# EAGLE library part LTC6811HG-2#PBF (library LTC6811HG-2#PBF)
Multicell Battery Balancer Automotive 48-Pin SSOP Tube Source: Datasheet
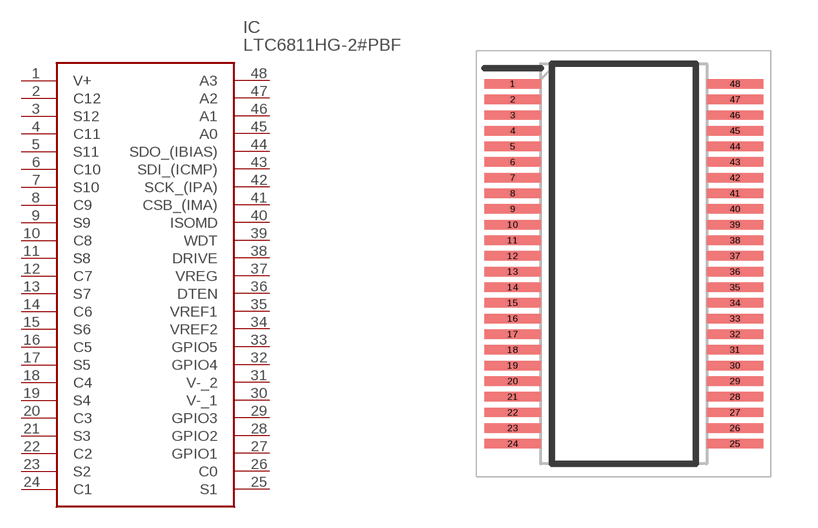
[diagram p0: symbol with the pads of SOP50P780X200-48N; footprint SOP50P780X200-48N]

Designator prefix IC

## LTC6811HG-2#PBF (Description: Multicell Battery Balancer Automotive 48-Pin SSOP Tube; Height: 2mm; Manufacturer_Name: Analog Devices; Manufacturer_Part_Number: LTC6811HG-2#PBF; Mouser_Part_Number: 584-LTC6811HG-2#PBF; Mouser_Price-Stock: https://www.mouser.co.uk/ProductDetail/Analog-Devices/LTC6811HG-2PBF?qs=oahfZPh6IAIAIIgZWv9WxQ%3D%3D)  [SOP50P780X200-48N]
1  V+
2  C12
3  S12
4  C11
5  S11
6  C10
7  S10
8  C9
9  S9
10  C8
11  S8
12  C7
13  S7
14  C6
15  S6
16  C5
17  S5
18  C4
19  S4
20  C3
21  S3
22  C2
23  S2
24  C1
25  S1
26  C0
27  GPIO1
28  GPIO2
29  GPIO3
30  V-_1
31  V-_2
32  GPIO4
33  GPIO5
34  VREF2
35  VREF1
36  DTEN
37  VREG
38  DRIVE
39  WDT
40  ISOMD
41  CSB_(IMA)
42  SCK_(IPA)
43  SDI_(ICMP)
44  SDO_(IBIAS)
45  A0
46  A1
47  A2
48  A3

## Footprint SOP50P780X200-48N (pad centres in mm)
48-Lead Plastic SSOP (5.3mm)
smd 1.8 x 0.3: 1 -3.55,5.75; 2 -3.55,5.25; 3 -3.55,4.75; 4 -3.55,4.25; 5 -3.55,3.75; 6 -3.55,3.25; 7 -3.55,2.75; 8 -3.55,2.25; 9 -3.55,1.75; 10 -3.55,1.25; 11 -3.55,0.75; 12 -3.55,0.25; 13 -3.55,-0.25; 14 -3.55,-0.75; 15 -3.55,-1.25; 16 -3.55,-1.75; 17 -3.55,-2.25; 18 -3.55,-2.75; 19 -3.55,-3.25; 20 -3.55,-3.75; 21 -3.55,-4.25; 22 -3.55,-4.75; 23 -3.55,-5.25; 24 -3.55,-5.75; 25 3.55,-5.75; 26 3.55,-5.25; 27 3.55,-4.75; 28 3.55,-4.25; 29 3.55,-3.75; 30 3.55,-3.25; 31 3.55,-2.75; 32 3.55,-2.25; 33 3.55,-1.75; 34 3.55,-1.25; 35 3.55,-0.75; 36 3.55,-0.25; 37 3.55,0.25; 38 3.55,0.75; 39 3.55,1.25; 40 3.55,1.75; 41 3.55,2.25; 42 3.55,2.75; 43 3.55,3.25; 44 3.55,3.75; 45 3.55,4.25; 46 3.55,4.75; 47 3.55,5.25; 48 3.55,5.75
